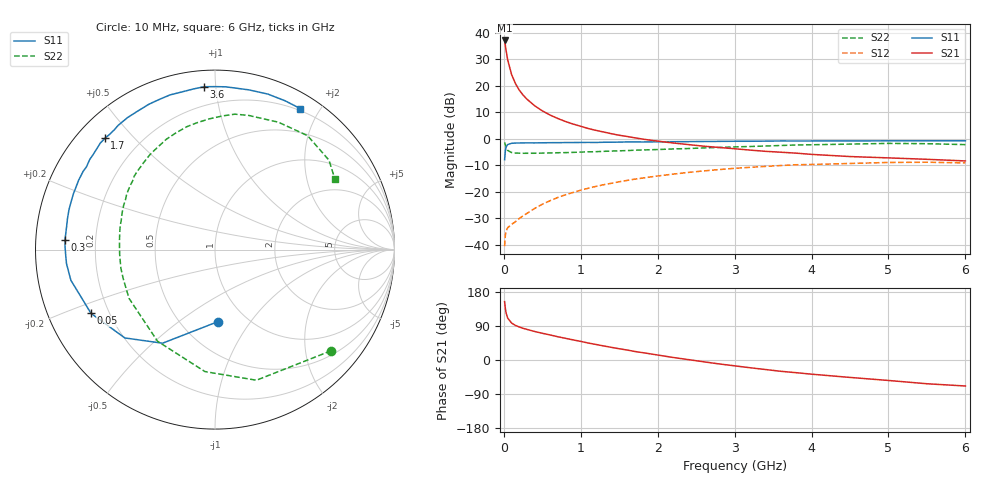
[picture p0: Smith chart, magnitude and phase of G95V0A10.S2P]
! SIEMENS Small Signal Semiconductors
! BFG235
! Si NPN RF Bipolar Junction Transistor in SOT223
! VCE = 5 V  IC = 100 mA
! Common Emitter S-Parameters:  July  1994
# GHz  S  MA  R  50
!  f  S11  S21  S12  S22
! GHz  MAG  ANG  MAG  ANG  MAG  ANG  MAG  ANG
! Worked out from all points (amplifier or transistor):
!   40 points, 10 MHz to 6 GHz, reference 50 ohm
!   highest |S21| = 37.2 dB at 10 MHz (marker M1)
!   |S21| within 3 dB of that: start of sweep to 25.43 MHz
!   unconditionally stable (mu >= 1): 471.5 MHz to 1.447 GHz
!   at 200 MHz: K = 0.77, MSG = 24.3 dB, |S12| = -30.2 dB
!   at 1.5 GHz: K = 0.99, MSG = 8.8 dB, |S12| = -16.3 dB
!   at 6 GHz: K = 0.90, MSG = 0.4 dB, |S12| = -9.1 dB
!   S11 on the Smith chart (normalised r, x): 10 MHz: 0.74, -0.71; 50 MHz: 0.13, -0.24; 300 MHz: 0.09, +0.03; 1.7 GHz: 0.08, +0.42; 3.6 GHz: 0.09, +0.93; 6 GHz: 0.18, +1.76
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0.01  0.4023 -87.9  72.46 154.0  0.0093 64.8  0.8577 -41.1
0.02  0.5982 -119.3  58.04 135.5  0.0151 51.5  0.7635 -72.4
0.03  0.7033 -135.6  46.24 123.5  0.018 42.2  0.682 -94.7
0.05  0.7768 -152.8  31.15 110.5  0.0208 34.3  0.6026 -122.1
0.1  0.821 -168.0  16.56 97.7  0.024 34.8  0.5507 -150.4
0.15  0.831 -174.6  11.14 91.3  0.0269 40.6  0.5365 -162.2
0.2  0.8326 -178.1  8.345 87.2  0.031 44.9  0.5346 -168.9
0.25  0.8359 178.6  6.722 83.6  0.0349 48.7  0.5317 -173.5
0.3  0.8377 176.3  5.618 80.8  0.0387 52.0  0.5319 -177.2
0.4  0.8364 171.6  4.225 75.3  0.0481 54.6  0.5326 177.6
0.5  0.84 168.0  3.373 70.5  0.0577 56.6  0.5355 173.3
0.6  0.8434 164.8  2.818 66.2  0.0673 56.8  0.5397 169.5
0.8  0.8479 158.4  2.126 57.3  0.0872 55.6  0.5472 162.7
1.1  0.8542 149.4  1.559 44.6  0.1161 51.3  0.5662 153.8
1.4  0.8609 142.1  1.246 33.3  0.1442 45.8  0.5858 145.6
1.7  0.8722 134.7  1.044 22.6  0.1721 39.7  0.6079 137.8
2.2  0.8823 123.5  0.833 6.7  0.2145 28.7  0.6421 124.2
3.2  0.8975 102.0  0.611 -20.4  0.2884 5.6  0.7142 98.0
3.6  0.9094 93.8  0.557 -29.8  0.3117 -4.4  0.7462 86.7
4.5  0.9098 78.0  0.461 -46.0  0.3412 -24.4  0.7929 63.5
5.5  0.9165 64.7  0.409 -62.7  0.3599 -46.5  0.8072 38.1
6  0.9181 58.8  0.381 -68.6  0.3495 -54.8  0.7753 30.6
